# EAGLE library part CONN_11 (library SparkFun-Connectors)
Multi connection point. Often used as Generic Header-pin footprint for 0.1 inch spaced/style header connections On any of the 0.1 inch spaced packages, you can populate with these: Break Away Headers - Straight (PRT-00116) Break Away Male Headers - Right Angle (PRT-00553) Female Headers (PRT-00115) Break Away Headers - Machine Pin (PRT-00117) Break Away Female Headers - Swiss Machine Pin (PRT-00743) For SCREWTERMINALS and SPRING TERMINALS visit here: Screw Terimnals on SparkFun.com (5mm/3.5mm/2.54mm spacing) This device is also useful as a general connection point to wire up your design to another part of your project. Our various solder wires solder well into these plated through hole pads. Hook-Up Wire - Assortment (Stranded, 22 AWG) (PRT-11375) Hook-Up Wire - Assortment (Solid Core, 22 AWG) (PRT-11367) View the entire wire category on our website here
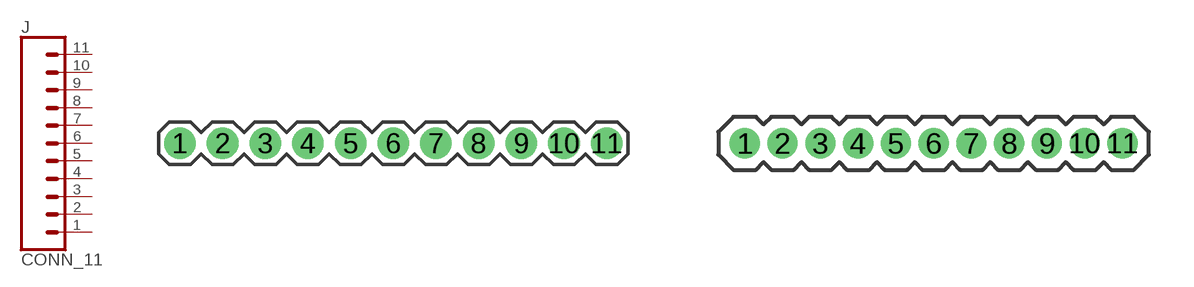
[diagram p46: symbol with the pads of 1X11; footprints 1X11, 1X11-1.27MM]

Designator prefix J

## CONN_11  [1X11]
1  1  pas
2  2  pas
3  3  pas
4  4  pas
5  5  pas
6  6  pas
7  7  pas
8  8  pas
9  9  pas
10  10  pas
11  11  pas

## CONN_11_1.27MM  [1X11-1.27MM]
Pads as for 1X11

## CONN_11LOCK  [1X11_LOCK]
Pads as for 1X11

## CONN_11LOCK_LONGPADS  [1X11_LOCK_LONGPADS]
Pads as for 1X11

## CONN_11LONGPADS  [1X11_LONGPADS]
Pads as for 1X11

## CONN_11POGOPIN_HOLES_ONLY  [1X11_HOLES_ONLY]
Pads as for 1X11

## CONN_111X11_NO_SILK  [1X11_NO_SILK]
Pads as for 1X11

## CONN_111X11_NO_SILK_KIT  [1X11_NO_SILK_KIT]
Pads as for 1X11

## Footprint 1X11 (pad centres in mm)
Plated Through Hole -11 Pin Specifications: Pin count:11 Pin pitch:0.1" Example device(s): CONN_11
drill 1.016 pad 1.88: 1 0,0; 2 2.54,0; 3 5.08,0; 4 7.62,0; 5 10.16,0; 6 12.7,0; 7 15.24,0; 8 17.78,0; 9 20.32,0; 10 22.86,0; 11 25.4,0

## Footprint 1X11-1.27MM (pad centres in mm)
Plated Through Hole -11 Pin 1.27mm Specifications: Pin count:11 Pin pitch:1.27mm Example device(s): CONN_11
drill 0.508 pad 1: 1 0,0; 2 1.27,0; 3 2.54,0; 4 3.81,0; 5 5.08,0; 6 6.35,0; 7 7.62,0; 8 8.89,0; 9 10.16,0; 10 11.43,0; 11 12.7,0

## Footprint 1X11_LOCK (pad centres in mm)
Plated Through Hole -11 Pin Locking Footprint Holes are offset 0.005" to hold pins in place while soldering. Specifications: Pin count:11 Pin pitch:0.1" Example device(s): CONN_11
drill 1.016 pad 1.88: 1 0,0.127; 2 2.54,-0.127; 3 5.08,0.127; 4 7.62,-0.127; 5 10.16,0.127; 6 12.7,-0.127; 7 15.24,0.127; 8 17.78,-0.127; 9 20.32,0.127; 10 22.86,-0.127; 11 25.4,0.127

## Footprint 1X11_LOCK_LONGPADS (pad centres in mm)
Plated Through Hole -11 Pin Locking Footprint w/ Long Pads Holes are offset 0.005" to hold pins in place while soldering. Specifications: Pin count:11 Pin pitch:0.1" Example device(s): CONN_11
drill 1.016 long: 1 0,0.127; 2 2.54,-0.127; 3 5.08,0.127; 4 7.62,-0.127; 5 10.16,0.127; 6 12.7,-0.127; 7 15.24,0.127; 8 17.78,-0.127; 9 20.32,0.127; 10 22.86,-0.127; 11 25.4,0.127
